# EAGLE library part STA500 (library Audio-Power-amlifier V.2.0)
STA500 is 30V 3.5A QUAD POWER HALF BRIDGE a monolithic quad half bridge stage in Multipower BCD Technology. The device can be used as dual bridge or reconfigured, by connecting CONFIG pin to Vdd pin, as single bridge with double current capability.
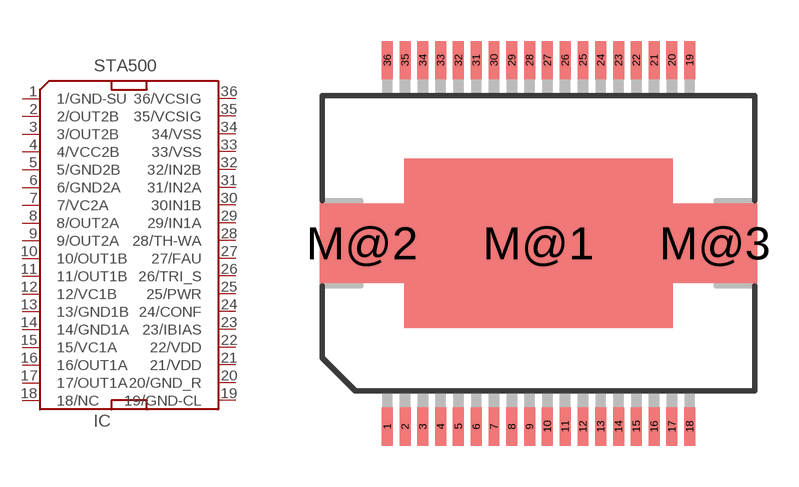
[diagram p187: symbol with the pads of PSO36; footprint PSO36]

Designator prefix IC

## STA500  [PSO36]
1  1/GND-SU  pwr
2  2/OUT2B  out
3  3/OUT2B  out
4  4/VCC2B  pwr
5  5/GND2B  pwr
6  6/GND2A  pwr
7  7/VC2A  pwr
8  8/OUT2A  out
9  9/OUT2A  out
10  10/OUT1B  out
11  11/OUT1B  out
12  12/VC1B  pwr
13  13/GND1B  pwr
14  14/GND1A  pwr
15  15/VC1A  pwr
16  16/OUT1A  out
17  17/OUT1A  out
18  18/NC  nc
19  19/GND-CL  pwr
20  20/GND_R  pwr
21  21/VDD  pwr
22  22/VDD  pwr
23  23/IBIAS
24  24/CONF
25  25/PWR  in
26  26/TRI_S  in
27  27/FAU  oc
28  28/TH-WA  oc
29  29/IN1A  in
30  30IN1B  in
31  31/IN2A  in
32  32/IN2B  in
33  33/VSS  pwr
34  34/VSS  pwr
35  35/VCSIG  pwr
36  36/VCSIG  pwr

## Footprint PSO36 (pad centres in mm)
36 LEADS POWER SMALL OUTLINE PACKAGE Source: http://www.st.com/stonline/books/pdf/docs/9426.pdf
smd 0.4 x 1.4: 1 -5.525,-6.7; 2 -4.875,-6.7; 3 -4.225,-6.7; 4 -3.575,-6.7; 5 -2.925,-6.7; 6 -2.275,-6.7; 7 -1.625,-6.7; 8 -0.975,-6.7; 9 -0.325,-6.7; 10 0.325,-6.7; 11 0.975,-6.7; 12 1.625,-6.7; 13 2.275,-6.7; 14 2.925,-6.7; 15 3.575,-6.7; 16 4.225,-6.7; 17 4.875,-6.7; 18 5.525,-6.7; 19 5.525,6.7; 20 4.875,6.7; 21 4.225,6.7; 22 3.575,6.7; 23 2.925,6.7; 24 2.275,6.7; 25 1.625,6.7; 26 0.975,6.7; 27 0.325,6.7; 28 -0.325,6.7; 29 -0.975,6.7; 30 -1.625,6.7; 31 -2.275,6.7; 32 -2.925,6.7; 33 -3.575,6.7; 34 -4.225,6.7; 35 -4.875,6.7; 36 -5.525,6.7
smd 9.8 x 6.2: M@1 0,0
smd 3.1 x 2.9: M@2 -6.45,0; M@3 6.45,0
